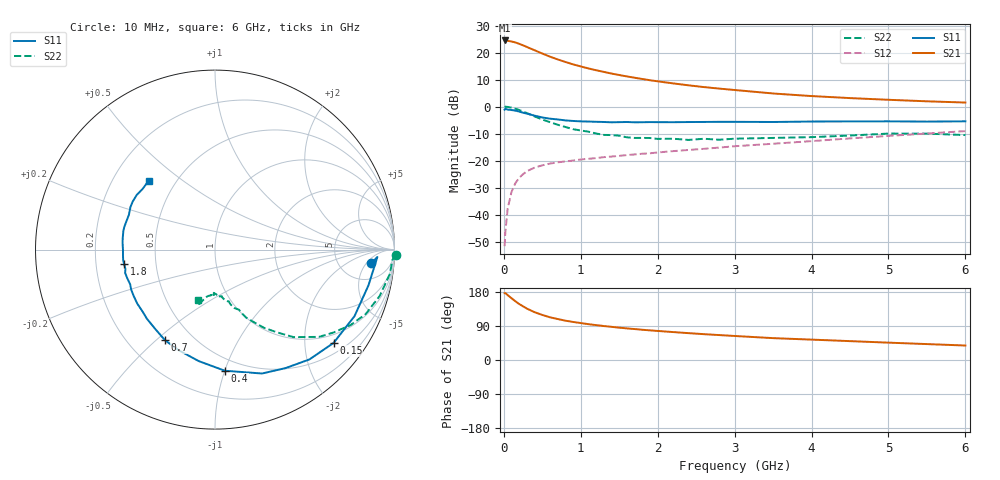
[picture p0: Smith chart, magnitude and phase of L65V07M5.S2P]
!  INFINEON TECHNOLOGIES Small Signal Semiconductors
! BFR380L3 , Si-NPN RF-Transistor in TSLP-3-1
!  Vce=5 V,  Ic=7.5 mA
! Common Emitter S-Parameters:  07. March 2005
#  GHz  S  MA  R  50
! f  S11  S21  S12  S22
! GHz  Mag  Ang  Mag  Ang  Mag  Ang  Mag  Ang
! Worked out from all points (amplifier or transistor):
!   36 points, 10 MHz to 6 GHz, reference 50 ohm
!   highest |S21| = 24.5 dB at 10 MHz (marker M1)
!   |S21| within 3 dB of that: start of sweep to 347.5 MHz
!   unconditionally stable (mu >= 1): 2.636 GHz to 4.61 GHz
!   at 250 MHz: K = 0.19, MSG = 23.9 dB, |S12| = -25.1 dB
!   at 1.4 GHz: K = 0.79, MSG = 15.4 dB, |S12| = -18.5 dB
!   at 6 GHz: K = 0.94, MSG = 5.3 dB, |S12| = -9.1 dB
!   S11 on the Smith chart (normalised r, x): 10 MHz: 10, -7; 150 MHz: 0.76, -2.70; 400 MHz: 0.40, -1.00; 700 MHz: 0.35, -0.54; 1.8 GHz: 0.32, -0.07; 6 GHz: 0.35, +0.38
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0.01  0.874 -5.0  16.72 176.4  0.0026 77.8  1.01 -1.6
0.02  0.9057 -2.6  16.64 176.6  0.0048 83.8  0.9903 -3.3
0.05  0.878 -13.1  16.5 171.2  0.013 84.5  0.9834 -8.0
0.1  0.8612 -25.5  15.99 163.0  0.0263 77.1  0.9533 -15.7
0.15  0.8407 -38.2  15.37 155.0  0.0381 71.2  0.9132 -23.2
0.2  0.807 -49.3  14.49 147.7  0.0481 66.3  0.8643 -29.1
0.25  0.7685 -59.2  13.59 141.6  0.0559 61.8  0.8057 -35.0
0.3  0.7384 -69.2  12.64 135.6  0.0637 58.0  0.7566 -40.0
0.4  0.6774 -85.3  11.01 126.1  0.074 52.2  0.6551 -48.1
0.5  0.6278 -98.3  9.575 118.9  0.0816 49.1  0.5755 -53.2
0.6  0.5959 -110.0  8.376 112.7  0.0879 47.1  0.5132 -58.0
0.7  0.5769 -118.8  7.446 108.1  0.0926 45.8  0.4603 -61.7
0.9  0.5405 -134.7  6.035 100.4  0.1 45.1  0.3808 -67.4
1.1  0.5273 -145.2  5.076 94.5  0.1078 45.8  0.3421 -71.8
1.4  0.5106 -157.8  4.074 87.5  0.1186 47.1  0.2963 -76.3
1.8  0.5122 -170.8  3.235 79.8  0.1337 49.8  0.2625 -82.6
2.2  0.5128 -179.9  2.683 73.7  0.1494 52.3  0.2536 -87.0
2.8  0.5211 168.3  2.148 65.8  0.1739 55.5  0.2429 -94.5
3.5  0.5175 157.9  1.745 57.7  0.2047 57.2  0.2624 -98.9
4.5  0.531 149.7  1.433 49.8  0.2569 59.8  0.2905 -103.5
5.5  0.5263 140.0  1.25 42.0  0.3167 59.2  0.3152 -107.4
6  0.5324 134.0  1.185 38.2  0.3508 58.2  0.2963 -109.0
